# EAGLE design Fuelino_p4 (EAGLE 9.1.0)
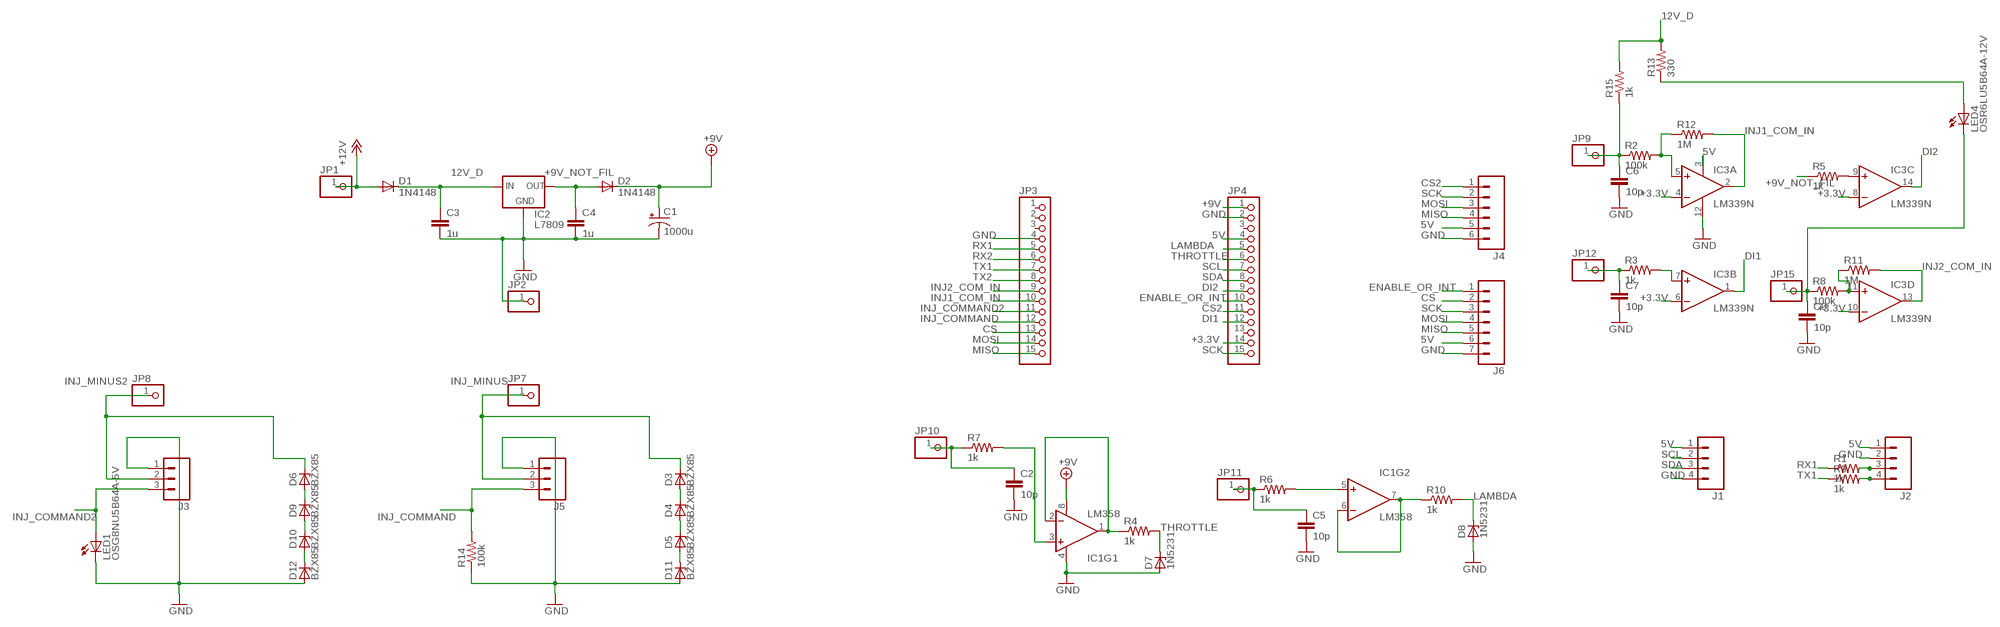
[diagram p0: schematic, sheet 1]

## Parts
C1  1000u  CAP_POLPTH4  [CPOL-RADIAL-1000UF-25V]
C2  10p  C2.5/2  [C2.5-2]
C3  1u  C2.5/2  [C2.5-2]
C4  1u  C2.5/2  [C2.5-2]
C5  10p  C2.5/2  [C2.5-2]
C6  10p  C2.5/2  [C2.5-2]
C7  10p  C2.5/2  [C2.5-2]
C9  10p  C2.5/2  [C2.5-2]
D1  1N4148  1N4148DO35-7  [DO35-7]
D2  1N4148  1N4148DO35-7  [DO35-7]
D3  BZX85  [DO41Z10]
D4  BZX85  [DO41Z10]
D5  BZX85  [DO41Z10]
D6  BZX85  [DO41Z10]
D7  1N5231  ZENER-DIODEZD-5  [ZDIO-5]
D8  1N5231  ZENER-DIODEZD-5  [ZDIO-5]
D9  BZX85  [DO41Z10]
D10  BZX85  [DO41Z10]
D11  BZX85  [DO41Z10]
D12  BZX85  [DO41Z10]
IC1  LM358  [DIP08]
IC2  L7809  78XXS  [78XXS]
IC3  LM339N  [DIL14]
J1  M04PTH  [1X04]
J2  M04PTH  [1X04]
J3  M03PTH  [1X03]
J4  M06SILK_FEMALE_PTH  [1X06]
J5  M03PTH  [1X03]
J6  M07  [1X07]
JP1  PINHD-1X1  [1X01]
JP2  PINHD-1X1  [1X01]
JP3  PINHD-1X15  [1X15]
JP4  PINHD-1X15  [1X15]
JP7  PINHD-1X1  [1X01]
JP8  PINHD-1X1  [1X01]
JP9  PINHD-1X1  [1X01]
JP10  PINHD-1X1  [1X01]
JP11  PINHD-1X1  [1X01]
JP12  PINHD-1X1  [1X01]
JP15  PINHD-1X1  [1X01]
LED1  OSG8NU5B64A-5V  LED5MM  [LED5MM]
LED4  OSR6LU5B64A-12V  LED5MM  [LED5MM]
R1  1k  R-US_0204/5  [0204/5]
R2  100k  R-US_0204/5  [0204/5]
R3  1k  R-US_0204/5  [0204/5]
R4  1k  R-US_0204/5  [0204/5]
R5  1k  R-US_0204/5  [0204/5]
R6  1k  R-US_0204/5  [0204/5]
R7  1k  R-US_0204/5  [0204/5]
R8  100k  R-US_0204/5  [0204/5]
R9  1k  R-US_0204/5  [0204/5]
R10  1k  R-US_0204/5  [0204/5]
R11  1M  R-US_0204/5  [0204/5]
R12  1M  R-US_0204/5  [0204/5]
R13  330  R-US_0204/5  [0204/5]
R14  100k  R-US_0204/5  [0204/5]
R15  1k  R-US_0204/5  [0204/5]

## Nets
5V: IC3.3(P:V+) J1.1 J2.1 J4.5 J6.6 JP4.4
12V_D: C3.1 D1.C IC2.IN R13.2 R15.2
+3.3V: IC3.4(A:-IN) IC3.6(B:-IN) IC3.8(C:-IN) IC3.10(D:-IN) JP4.14
+9V: C1.+ D2.C IC1.8(V+) JP4.1
+9V_NOT_FIL: C4.1 D2.A IC2.OUT R5.1
+12V: D1.A JP1.1
CS: J6.2 JP3.13
CS2: J4.1 JP4.11
DI1: IC3.1(B:OUT) JP4.12
DI2: IC3.14(C:OUT) JP4.9
ENABLE_OR_INT: J6.1 JP4.10
GND: C1.- C2.2 C3.2 C4.2 C5.2 C6.2 C7.2 C9.2 D7.A D8.A D11.A D12.A IC1.4(V-) IC2.GND IC3.12(P:GND) J1.4 J2.2 J3.1 J4.6 J5.1 J6.7 JP2.1 JP3.4 JP4.2 LED1.K(C) R14.1
INJ1_COM_IN: IC3.2(A:OUT) JP3.10 R12.2
INJ2_COM_IN: IC3.13(D:OUT) JP3.9 R11.2
INJ_COMMAND: J5.3 JP3.12 R14.2
INJ_COMMAND2: J3.3 JP3.11 LED1.A
INJ_MINUS: D3.C J5.2 JP7.1
INJ_MINUS2: D6.C J3.2 JP8.1
LAMBDA: D8.C JP4.5 R10.2
MISO: J4.4 J6.5 JP3.15
MOSI: J4.3 J6.4 JP3.14
N$1: D6.A D9.C
N$2: D9.A D10.C
N$3: D3.A D4.C
N$4: D4.A D5.C
N$5: D10.A D12.C
N$6: D5.A D11.C
N$7: IC3.9(C:+IN) R5.2
N$8: IC3.11(D:+IN) R8.2 R11.1
N$9: C6.1 JP9.1 R2.1 R15.1
N$10: IC3.5(A:+IN) R2.2 R12.1
N$11: C7.1 JP12.1 R3.1
N$12: IC3.7(B:+IN) R3.2
N$13: IC1.1(OUT) IC1.2(-IN) R4.1
N$14: J2.3 R1.2
N$15: LED4.A R13.1
N$16: C9.1 JP15.1 LED4.K(C) R8.1
N$18: J2.4 R9.2
N$38: C5.1 JP11.1 R6.1
N$39: IC1.5(+IN) R6.2
N$41: IC1.6(-IN) IC1.7(OUT) R10.1
N$44: C2.1 JP10.1 R7.1
N$46: IC1.3(+IN) R7.2
RX1: JP3.5 R1.1
RX2: JP3.6
SCK: J4.2 J6.3 JP4.15
SCL: J1.2 JP4.7
SDA: J1.3 JP4.8
THROTTLE: D7.C JP4.6 R4.2
TX1: JP3.7 R9.1
TX2: JP3.8
Unconnected: JP3.1 JP3.2 JP3.3 JP4.3 JP4.13

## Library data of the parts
C1 = SparkFun-Capacitors:CAP_POL: Capacitor Polarized
C2-C7 C9 = capacitor-wima:C: CAPACITOR
D1 D2 = diode:1N4148: DIODE
D3-D6 D9-D12 = diode:BZX85: Z DIODE
D7 D8 = diode:ZENER-DIODE: Z-Diode
IC1 = SparkFun-AnalogIC:LM358: Jellybean op-amp; PROD_ID: IC-09172
IC2 = v-reg:78XXS: VOLTAGE REGULATOR
IC3 = linear:LM339: Low Power Low Offset Voltage Quad Comparators with open collector; LM139/LM239/LM339/LM2901/LM3302
J1 J2 = SparkFun-Connectors:M04: Header 4 Standard 4-pin 0.1" header. Use with straight break away headers (SKU : PRT-00116), right angle break away headers (PRT-00553), swiss pins (PRT-00743), machine pins (PRT-00117), and female headers (PRT-00115). Molex polarized connector foot print use with SKU : PRT-08231 with associated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; PROD_ID: CONN-09696
J3 J5 = SparkFun-Connectors:M03: Header 3 Standard 3-pin 0.1" header. Use with straight break away headers (SKU : PRT-00116), right angle break away headers (PRT-00553), swiss pins (PRT-00743), machine pins (PRT-00117), and female headers (PRT-00115). Molex polarized connector foot print use with SKU : PRT-08232 with associated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
J4 = SparkFun-Connectors:M06: Header 6 Standard 6-pin 0.1" header. Use with straight break away headers (SKU : PRT-00116), right angle break away headers (PRT-00553), swiss pins (PRT-00743), machine pins (PRT-00117), and female headers (PRT-00115). Molex polarized connector foot print use with SKU : PRT-08094 with associated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; PROD_ID: CONN-08437
J6 = SparkFun-Connectors:M07: Header 7 Standard 7-pin 0.1" header. Use with straight break away headers (SKU : PRT-00116), right angle break away headers (PRT-00553), swiss pins (PRT-00743), machine pins (PRT-00117), and female headers (PRT-00115). NOTES ON THE VARIANTS LOCK and LOCK_LONGPADS... This footprint was designed to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
JP1 JP2 JP7-JP12 JP15 = pinhead:PINHD-1X1: PIN HEADER
JP3 JP4 = pinhead:PINHD-1X15: PIN HEADER
LED1 LED4 = led:LED: LED
R1-R15 = resistor:R-US_: RESISTOR, American symbol

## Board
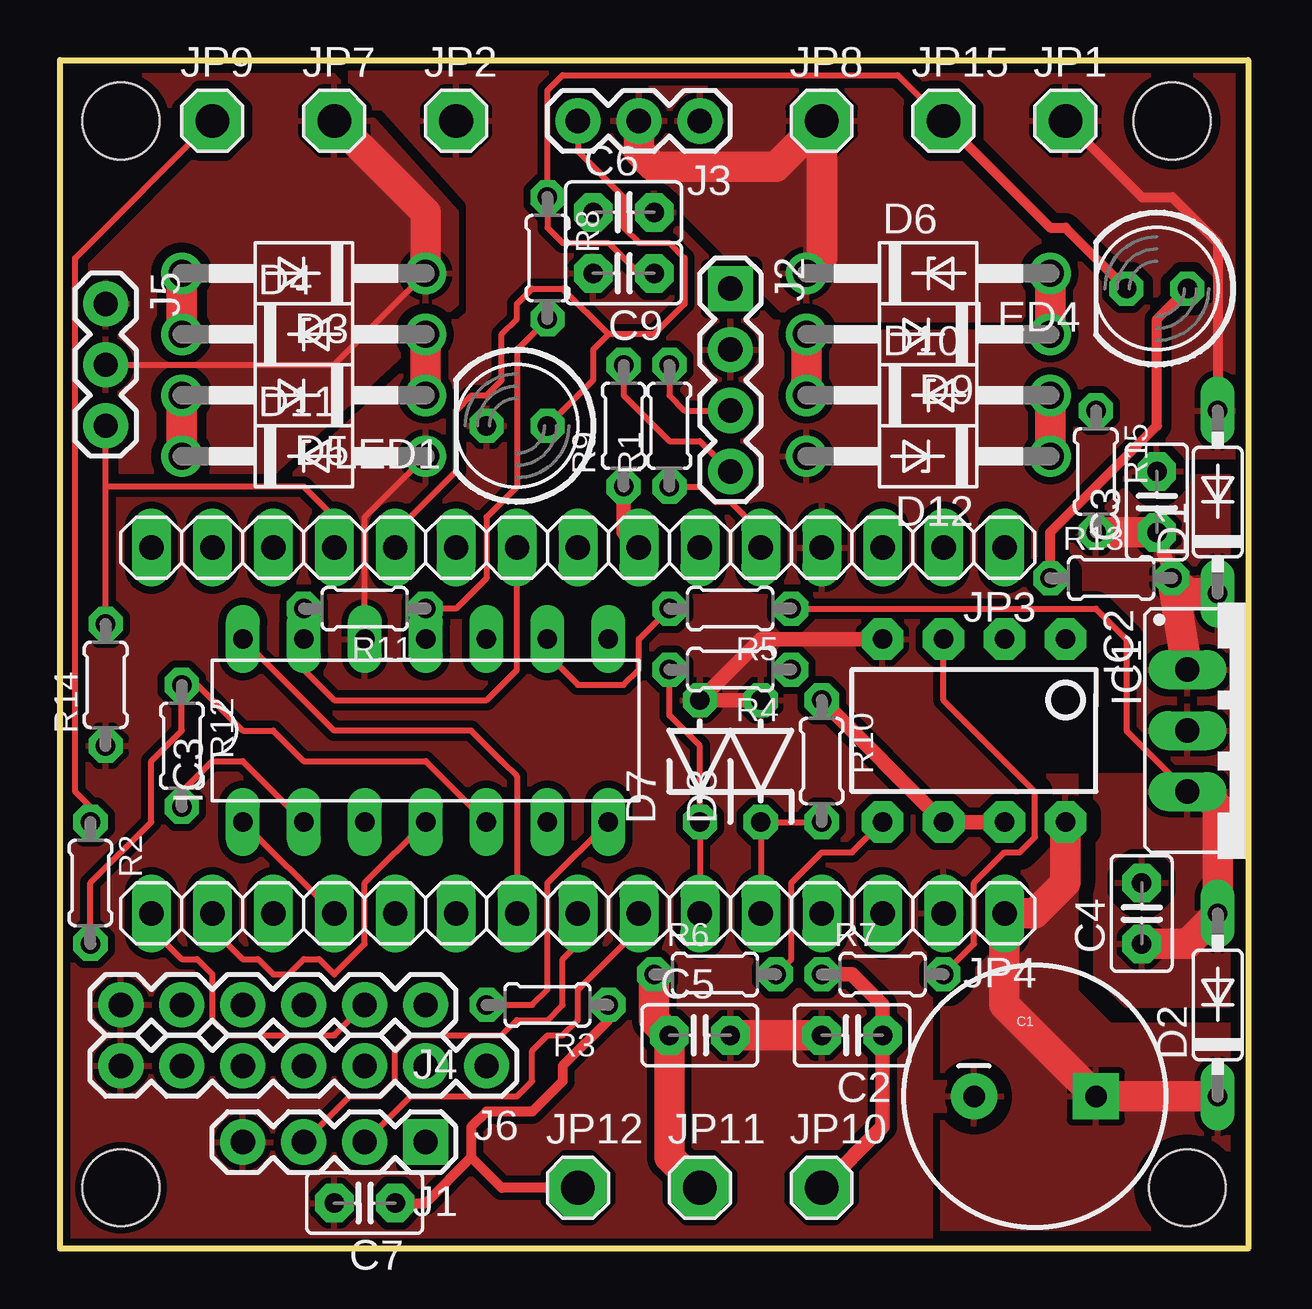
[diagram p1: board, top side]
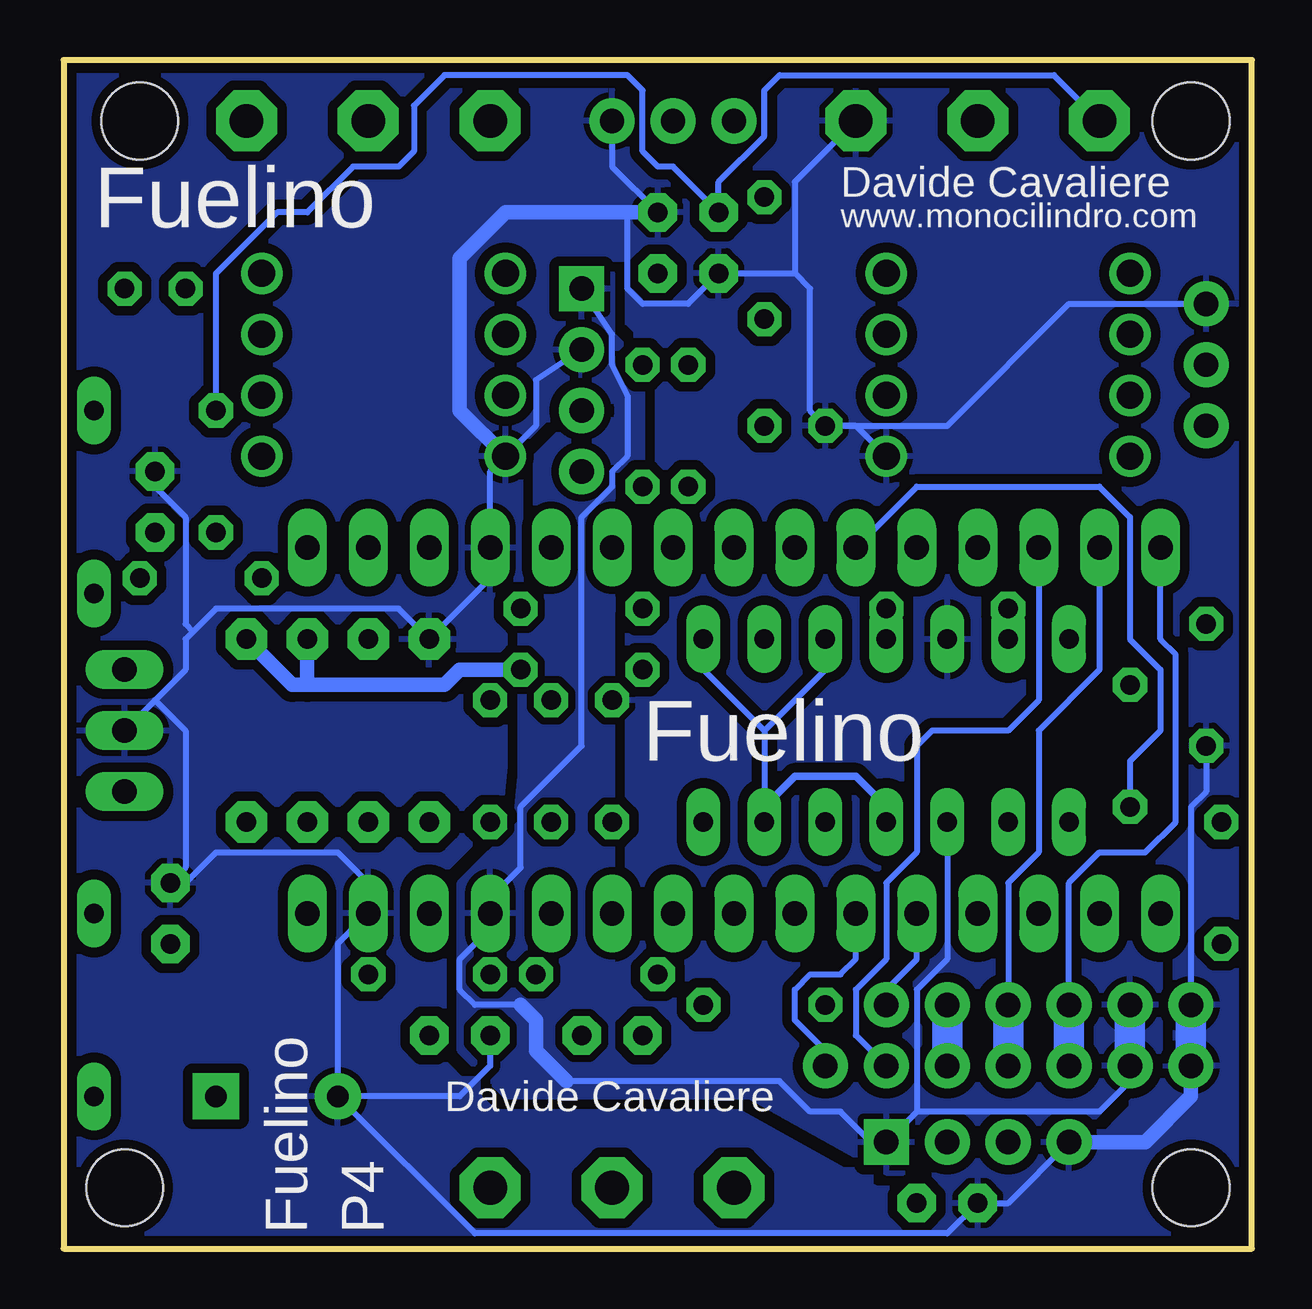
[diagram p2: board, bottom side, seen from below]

Size 49.53 x 49.53 mm. Coordinates in mm from the lower left corner, seen from the top.
Outline: 0,0 49.2,0
Outline: 0,0 49.53,0 49.53,49.53 0,49.53 0,0
Copper layers (1*16): Top 0.035mm / dielectric 1.5mm / Bottom 0.035mm
Design rules "SparkFun": minimum track width 8mil, minimum drill 20mil, track to track 8mil, track to pad 8mil, pad to pad 8mil, via to via 8mil, smd to smd 8mil, copper to edge 8mil, drill to drill 8mil, minimum pad ring 12mil, minimum via ring 10mil, stop-mask expansion 4mil, vias tented up to drill 20mil, thermal gap 10mil
Holes 3.2 mm at 2.54,46.99 2.54,2.54 46.99,2.54 46.35,46.99

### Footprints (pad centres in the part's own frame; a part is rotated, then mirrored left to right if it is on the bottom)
CPOL-RADIAL-1000UF-25V = drill 0.9 pad 1.93 square: + 2.54,0 | drill 0.9 pad 1.93: - -2.54,0
C2.5-2 = drill 0.813 pad 1.6 octagon: 1 -1.27,0; 2 1.27,0
DO35-7 = drill 0.813 long: A 3.81,0; C -3.81,0
DO41Z10 = drill 1.118: A 5.08,0; C -5.08,0
ZDIO-5 = drill 0.813 octagon: A 2.54,0; C -2.54,0
DIP08 = drill 0.813 pad 1.727 octagon: 1 -3.81,-3.81; 2 -1.27,-3.81; 3 1.27,-3.81; 4 3.81,-3.81; 5 3.81,3.81; 6 1.27,3.81; 7 -1.27,3.81; 8 -3.81,3.81
78XXS = drill 1.016 long: GND 0,-2.54; IN -2.54,-2.54; OUT 2.54,-2.54
DIL14 = drill 0.813 long: 1 -7.62,-3.81; 2 -5.08,-3.81; 3 -2.54,-3.81; 4 0,-3.81; 5 2.54,-3.81; 6 5.08,-3.81; 7 7.62,-3.81; 8 7.62,3.81; 9 5.08,3.81; 10 2.54,3.81; 11 0,3.81; 12 -2.54,3.81; 13 -5.08,3.81; 14 -7.62,3.81
1X04 = drill 1.016 pad 1.88 square: 1 0,0 | drill 1.016 pad 1.88: 2 2.54,0; 3 5.08,0; 4 7.62,0
1X03 = drill 1.016 pad 1.88: 1 0,0; 2 2.54,0; 3 5.08,0
1X06 = drill 1.016 pad 1.88: 1 0,0; 2 2.54,0; 3 5.08,0; 4 7.62,0; 5 10.16,0; 6 12.7,0
1X07 = drill 1.016 pad 1.88: 1 0,0; 2 2.54,0; 3 5.08,0; 4 7.62,0; 5 10.16,0; 6 12.7,0; 7 15.24,0
1X01 = drill 1.4 pad 2.54 octagon: 1 0,0
1X15 = drill 1.016 long: 1 -17.78,0; 2 -15.24,0; 3 -12.7,0; 4 -10.16,0; 5 -7.62,0; 6 -5.08,0; 7 -2.54,0; 8 0,0; 9 2.54,0; 10 5.08,0; 11 7.62,0; 12 10.16,0; 13 12.7,0; 14 15.24,0; 15 17.78,0
LED5MM = drill 0.813 octagon: A -1.27,0; K 1.27,0
0204/5 = drill 0.813 octagon: 1 -2.54,0; 2 2.54,0

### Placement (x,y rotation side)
C1  40.64,6.35 0 top
C2  33.02,8.89 180 top
C3  45.72,31.11 90 top
C4  45.09,13.97 90 top
C5  26.67,8.89 0 top
C6  23.5,43.18 0 top
C7  12.7,1.91 180 top
C9  23.5,40.64 180 top
D1  48.26,31.11 90 top
D2  48.26,10.16 90 top
D3  10.16,40.64 180 top
D4  10.16,38.1 0 top
D5  10.16,35.56 180 top
D6  36.2,40.64 0 top
D7  26.67,20.32 90 top
D8  29.21,20.32 90 top
D9  36.2,38.1 180 top
D10  36.2,35.56 0 top
D11  10.16,33.02 0 top
D12  36.2,33.02 180 top
IC1  38.1,21.59 180 top
IC2  49.53,21.59 270 top
IC3  15.24,21.59 0 top
J1  15.24,4.45 180 top
J2  27.94,40.01 270 top
J3  26.67,46.99 180 top
J4  15.24,10.16 180 top
J5  1.91,39.37 270 top
J6  17.78,7.62 180 top
JP1  41.91,46.99 0 top
JP2  16.51,46.99 0 top
JP3  21.59,29.21 180 top
JP4  21.59,13.97 180 top
JP7  11.43,46.99 0 top
JP8  31.75,46.99 0 top
JP9  6.35,46.99 0 top
JP10  31.75,2.54 0 top
JP11  26.67,2.54 0 top
JP12  21.59,2.54 0 top
JP15  36.83,46.99 0 top
LED1  19.05,34.29 180 top
LED4  45.72,40.01 180 top
R1  25.4,34.29 90 top
R2  1.27,15.24 270 top
R3  20.32,10.16 180 top
R4  27.94,24.13 180 top
R5  27.94,26.67 180 top
R6  27.3,11.43 0 top
R7  34.29,11.43 0 top
R8  20.32,41.27 270 top
R9  23.5,34.29 90 top
R10  31.75,20.32 270 top
R11  12.7,26.67 180 top
R12  5.08,20.95 270 top
R13  43.81,27.94 0 top
R14  1.91,23.5 90 top
R15  43.18,32.38 270 top

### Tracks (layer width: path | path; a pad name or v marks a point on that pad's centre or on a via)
5V
  Bottom 0.254: 13.97,5.71 6.35,5.71 5.08,6.99 J6.6 | IC3.3 12.7,12.06 13.97,10.79 13.97,5.71 | 13.97,5.71 J1.1 15.88,4.45 17.14,5.71 18.41,5.71 19.68,6.99 28.57,6.99 | 30.48,10.16 32.38,10.16 33.02,10.79 33.02,12.06 31.75,13.34 JP4.4 31.75,14.61 30.48,15.88 30.48,18.41 27.94,20.95 27.94,30.48 26.67,31.75 26.67,32.38 26.04,33.02 26.04,35.56 26.67,36.83 26.67,38.1 J2.1
  Bottom 0.61: 30.48,10.16 29.84,9.53 29.84,8.26 28.57,6.99
  Bottom 1.27: J6.6 J4.5
  pour Bottom (isolate 0.406): 28.57,40.01 28.57,39.37 31.75,6.99 31.11,6.35 20.95,6.35 15.24,3.17 8.89,3.17 3.81,8.26 3.81,12.06 4.45,12.7 28.57,12.7 28.57,17.78 26.67,20.95 26.67,26.67 25.4,26.67 25.4,36.83
  pour Bottom (isolate 0.305): 31.75,6.99 33.02,8.26 33.02,15.24 30.48,17.78 30.48,27.3 29.84,30.48 29.84,31.75 29.84,33.02 28.57,34.29 28.57,40.64 26.67,40.64 26.67,14.61 26.67,6.99
12V_D
  Top 0.61: R13.2 C3.1
  Top 1.27: IC2.IN R13.2 46.99,27.3 D1.C | R15.2 C3.1
  pour Top (isolate 0.61, rank 3): 40.64,38.73 40.64,27.94 44.45,22.86 49.53,22.86 49.53,38.73
+3.3V
  Top 0.254: JP4.14 6.35,13.34 7.62,12.06 8.26,12.06 8.89,11.43 9.53,11.43 10.16,12.06 10.79,12.06 11.43,11.43 12.7,12.7 12.7,15.24 IC3.4
  Bottom 0.254: IC3.8 22.86,24.13 20.32,21.59 | 20.32,21.59 20.32,18.41 IC3.6 | IC3.10 17.78,24.13 20.32,21.59
  Bottom 0.305: IC3.4 15.24,18.41 16.51,19.68 19.05,19.68 20.32,18.41
+9V
  Top 1.27: D2.C C1.+ 39.37,10.16 JP4.1 40.64,13.97 41.91,15.24 IC1.8
  pour Top (isolate 0.61, rank 2): 40.64,19.68 49.53,19.68 49.53,0 36.83,0 36.83,15.88
+9V_NOT_FIL
  Top 0.254: R5.1 43.18,26.67 44.45,25.4 44.45,21.59 IC2.OUT
  Top 1.27: C4.1 46.99,12.7 D2.A 48.26,18.41 47.62,19.05 IC2.OUT
  pour Top (isolate 0.61): 43.18,19.68 43.18,11.43 44.45,10.16 49.53,10.16 49.53,19.68
+12V
  Top 0.406: JP1.1 45.09,43.81 46.35,43.81 48.26,41.91 D1.A
  pour Top (isolate 0.406, rank 2): 34.29,49.53 34.29,43.81 43.81,33.02 49.53,33.02 49.53,49.53
CS
  Bottom 0.254: JP3.13 8.89,22.86 10.16,21.59 13.34,21.59 13.97,20.95 13.97,16.51 15.24,15.24 15.24,12.06 16.51,10.79 16.51,8.89 J6.2
CS2
  Bottom 0.254: J4.1 15.24,10.79 13.97,12.06 JP4.11
DI1
  Top 0.254: IC3.1 JP4.12
DI2
  Top 0.254: IC3.14 11.43,21.59 17.14,21.59 18.41,20.32 19.05,19.68 JP4.9
ENABLE_OR_INT
  Bottom 0.254: J6.1 17.78,8.26 19.05,9.53 19.05,10.79 18.41,11.43 17.14,11.43 16.51,12.06 JP4.10
GND
  Top 0.254: IC3.12 12.7,30.48 D11.A
  Top 0.61: D8.A D7.A 29.21,25.4 IC1.4
  Top 1.27: C5.2 C2.2
  Bottom 0.254: C1.- 38.1,12.7 JP4.2 36.83,15.24 38.1,16.51 43.18,16.51 44.45,15.24 C4.2 44.45,15.88 44.45,21.59 45.72,22.86 | IC2.GND 45.72,22.86 | 44.13,25.72 43.18,26.67 35.56,26.67 IC1.4 31.75,27.94 JP3.4 31.75,32.38 D12.A 29.84,34.29 29.84,36.2 J2.2 | 44.13,25.72 44.45,25.4 44.45,24.13 45.72,22.86 | D11.A 16.51,34.29 LED1.K | LED1.K 12.7,34.29 7.62,39.37 J5.1 | R14.1 1.91,19.05 2.54,18.41 J4.6 | C1.- 32.38,0.64 12.7,0.64 C7.2 10.16,1.91 J1.4 | C2.2 31.75,7.62 33.02,6.35 C1.- | 44.13,25.72 44.45,26.04 44.45,30.48 45.72,31.75 C3.2 | J3.1 26.67,45.09 C6.2 | 26.04,43.18 26.04,40.01 25.4,39.37 23.5,39.37 C9.2 19.05,40.64 | LED1.K 18.41,34.92 18.41,40.01 19.05,40.64 | JP2.1 19.05,44.45 19.05,40.64
  Bottom 0.61: D12.A 33.02,34.92 33.02,41.27 31.11,43.18 26.04,43.18 C6.2 | J1.4 4.45,4.45 2.54,6.35 J6.7
  Bottom 1.27: J4.6 J6.7
  pour Bottom (isolate 0.406, rank 2): 0,49.53 49.53,49.53 49.53,0 0,0
  pour Top (isolate 0.305, rank 6): 0,49.53 49.53,49.53 49.53,0 0,0
INJ1_COM_IN
  Top 0.254: R12.2 5.08,19.05 6.35,20.32 7.62,20.32 IC3.2
  Bottom 0.254: JP3.10 13.97,31.75 6.35,31.75 5.08,30.48 5.08,25.4 3.81,24.13 3.81,21.59 5.08,20.32 R12.2
INJ2_COM_IN
  Top 0.254: R11.2 10.16,24.13 11.43,22.86 17.78,22.86 19.05,24.13 JP3.9
  Bottom 0.254: R11.2 IC3.13
INJ_COMMAND
  Top 0.254: 1.91,31.75 J5.3 | JP3.12 11.43,30.48 10.16,31.75 1.91,31.75 | R14.2 1.91,31.75
INJ_COMMAND2
  Top 0.254: J3.3 21.59,45.72 23.5,43.81 23.5,42.55 24.13,41.91 25.4,41.91 26.04,41.27 26.04,39.37 24.77,38.1 22.86,38.1 | 22.86,38.1 22.23,37.47 22.23,36.2 LED1.A | 13.97,29.84 16.51,32.38 16.51,34.92 17.14,35.56 17.78,35.56 18.41,36.2 18.41,38.1 19.05,38.73 19.05,39.37 19.68,40.01 20.95,40.01 22.86,38.1
  Top 0.406: 13.97,29.84 JP3.11
INJ_MINUS
  Top 0.254: J5.2 11.43,36.83 D3.C
  Top 1.27: D3.C 15.24,43.18 JP7.1
  pour Top (isolate 0.406, rank 5): 10.79,49.53 0,49.53 0,24.13 16.51,39.37 16.51,43.18
INJ_MINUS2
  Top 1.27: D6.C 31.75,41.27 JP8.1 29.84,45.09 24.77,45.09 24.13,45.72 J3.2
  pour Top (isolate 0.406): 19.68,49.53 30.48,38.73 45.72,38.73 34.29,49.53
LAMBDA
  Top 0.254: JP4.5 D8.C R10.2
MISO
  Bottom 0.254: J4.4 7.62,15.24 6.35,16.51 4.45,16.51 3.17,17.78 3.17,24.77 3.81,25.4 JP3.15
  Bottom 1.27: J6.5 J4.4
MOSI
  Bottom 0.254: JP3.14 6.35,24.13 8.89,21.59 8.89,16.51 10.16,15.24 J4.3
  Bottom 1.27: J6.4 J4.3
N$1
  Top 1.27: D6.A D9.C
N$2
  Top 1.27: D9.A D10.C
N$3
  Top 1.27: D3.A D4.C
N$4
  Top 1.27: D4.A D5.C
N$5
  Top 1.27: D10.A D12.C
N$6
  Top 1.27: D11.C D5.A
N$7
  Top 0.254: IC3.9 20.32,24.77 21.59,23.5 23.5,23.5 24.13,24.13 24.13,25.4 R5.2
N$8
  Top 0.254: R8.2 19.05,37.47 19.05,31.75 17.78,30.48 17.78,27.94 16.51,26.67 R11.1 IC3.11
N$9
  Top 0.254: R2.1 1.27,18.41 0.64,19.05 0.64,41.27 JP9.1
  Bottom 0.254: R15.1 43.18,40.64 40.64,43.18 39.37,43.18 37.47,45.09 35.56,45.09 34.92,45.72 34.92,47.62 33.66,48.9 26.04,48.9 25.4,48.26 25.4,45.72 24.77,45.09 24.13,45.09 C6.1 22.23,44.45 20.32,46.35 20.32,48.26 19.68,48.9 8.26,48.9 JP9.1
N$10
  Top 0.254: R2.2 1.27,15.24 3.81,17.78 3.81,20.32 5.08,21.59 R12.1 5.71,23.5 7.62,21.59 8.89,21.59 10.16,20.32 15.24,20.32 IC3.5
N$11
  Top 0.406: R3.1 22.86,9.53 20.95,7.62 20.95,6.99 19.68,5.71 17.78,5.71 17.14,5.08 17.14,3.81 | 17.14,3.81 15.24,1.91 C7.1 | JP12.1 18.41,2.54 17.14,3.81
N$12
  Top 0.254: R3.2 19.68,10.16 20.32,10.79 20.32,15.24 IC3.7
N$13
  Bottom 0.61: R4.1 33.02,24.13 33.66,23.5 39.37,23.5 | 39.37,23.5 40.01,23.5 IC1.1 | IC1.2 39.37,23.5
N$14
  Top 0.254: R1.2 25.4,35.56 26.04,34.92 J2.3
N$15
  Top 0.406: LED4.A 45.72,38.73 45.72,34.29 41.27,29.84 R13.1
N$16
  Top 0.254: JP15.1 34.92,48.9 20.95,48.9 20.32,48.26 R8.1 20.32,42.55 20.95,41.91 22.86,41.91 24.13,40.64 C9.1
  Top 0.406: JP15.1 41.27,42.55 41.91,42.55 LED4.K
N$18
  Top 0.254: R9.2 23.5,35.56 25.4,33.66 26.67,33.66 J2.4
N$38
  Top 1.27: R6.1 24.77,9.53 C5.1 25.4,3.81 JP11.1
N$39
  Top 0.254: IC1.5 33.02,16.51 31.75,16.51 30.48,15.24 30.48,12.06 R6.2
N$41
  Top 0.61: R10.1 IC1.6 IC1.7
N$44
  Top 0.61: R7.1 33.02,11.43 34.29,10.16 C2.1 34.29,5.08 JP10.1
N$46
  Top 0.254: R7.2 38.1,12.7 38.1,15.24 39.37,16.51 40.01,16.51 40.64,17.14 40.64,19.05 36.83,22.86 IC1.3
RX1
  Top 0.254: R1.1 26.67,31.75 27.3,31.11 27.94,31.11 29.21,29.84 JP3.5
SCK
  Top 0.254: JP4.15 3.81,13.34 5.08,12.06 5.71,12.06 6.35,11.43 6.35,9.53 6.99,8.89 11.43,8.89 J4.2
  Bottom 1.27: J6.3 J4.2
SCL
  Top 0.254: J1.2 14.61,6.35 19.05,6.35 19.68,6.99 19.68,8.26 20.32,8.89 20.95,8.89 21.59,9.53 21.59,10.79 24.13,13.34 JP4.7
SDA
  Top 0.254: J1.3 12.06,6.35 13.34,6.35 13.97,6.99 13.97,8.26 14.61,8.89 18.41,8.89 19.05,9.53 20.32,9.53 20.95,10.16 20.95,12.06 21.59,12.7 JP4.8
THROTTLE
  Top 0.254: JP4.6 D7.C 26.67,20.95 25.4,22.23 R4.2
TX1
  Top 0.61: R9.1 23.5,29.84 JP3.7

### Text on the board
bNames: Davide Cavaliere | www.monocilindro.com | Fuelino | Fuelino | Davide Cavaliere | P4 | Fuelino

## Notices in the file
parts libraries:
SparkFun-Capacitors: Licensing: Creative Commons ShareAlike 4.0 International - https://creativecommons.org/licenses/by-sa/4.0
